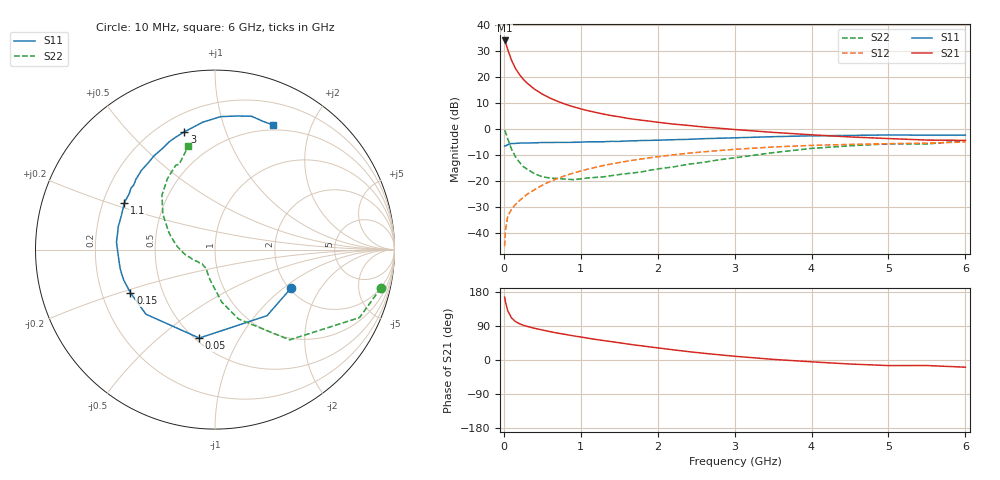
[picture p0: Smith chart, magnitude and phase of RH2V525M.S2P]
! SIEMENS Small Signal Semiconductors
! BFR106
! Si NPN RF Bipolar Junction Transistor in SOT23
! VCE = 2.5 V  IC = 25 mA
! Common Emitter S-Parameters:  August  1996
# GHz  S  MA  R  50
!  f  S11  S21  S12  S22
! GHz  MAG  ANG  MAG  ANG  MAG  ANG  MAG  ANG
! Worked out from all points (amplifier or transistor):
!   36 points, 10 MHz to 6 GHz, reference 50 ohm
!   highest |S21| = 34.2 dB at 10 MHz (marker M1)
!   |S21| within 3 dB of that: start of sweep to 45.07 MHz
!   unconditionally stable (mu >= 1): 324 MHz to 2.431 GHz; 5.267 GHz to end of sweep
!   at 250 MHz: K = 0.94, MSG = 22.9 dB, |S12| = -26.4 dB
!   at 1.4 GHz: K = 1.07, MAG = 7.7 dB, |S12| = -13.5 dB
!   at 6 GHz: K = 1.01, MAG = -0.2 dB, |S12| = -5.0 dB
!   S11 on the Smith chart (normalised r, x): 10 MHz: 2.04, -1.14; 50 MHz: 0.53, -0.69; 150 MHz: 0.32, -0.22; 1.1 GHz: 0.29, +0.22; 3 GHz: 0.30, +0.73; 6 GHz: 0.44, +1.48
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0.01  0.4745 -27.1  51.33 166.2  0.0055 84.5  0.9487 -13.0
0.02  0.4685 -51.8  47.52 154.8  0.0107 71.6  0.8899 -25.2
0.05  0.5006 -100.1  34.47 130.1  0.0206 58.2  0.6524 -50.4
0.1  0.527 -136.9  21.31 111.1  0.0285 53.6  0.4086 -71.2
0.15  0.5292 -152.9  14.9 101.6  0.0349 55.2  0.2949 -82.7
0.2  0.5363 -161.6  11.48 96.1  0.0411 58.2  0.2319 -88.5
0.25  0.5388 -168.0  9.223 91.8  0.0477 60.6  0.1905 -95.0
0.3  0.5384 -172.2  7.746 88.8  0.0548 62.8  0.1692 -99.6
0.4  0.5427 -179.3  5.88 83.6  0.068 65.3  0.1372 -107.6
0.5  0.5505 175.6  4.729 79.2  0.0826 66.3  0.1202 -113.5
0.6  0.5502 170.7  3.967 74.9  0.0972 66.6  0.1136 -118.3
0.7  0.554 166.8  3.427 70.9  0.1115 66.5  0.1113 -123.8
0.9  0.5552 159.9  2.703 63.9  0.1411 65.0  0.1059 -132.5
1.1  0.5688 152.7  2.252 57.3  0.1699 63.1  0.1142 -139.9
1.3  0.5704 146.9  1.941 51.2  0.1987 60.6  0.12 -147.4
1.6  0.5895 138.4  1.621 42.5  0.2396 56.5  0.1384 -157.8
2.2  0.6236 122.9  1.251 26.9  0.3181 47.5  0.1857 -177.4
3  0.678 104.6  0.981 9.9  0.4066 34.9  0.2788 158.5
3.5  0.7134 95.4  0.864 1.7  0.4518 27.2  0.3508 145.9
4.5  0.7542 80.7  0.705 -10.6  0.5059 12.3  0.4756 123.9
5.5  0.7629 69.3  0.614 -14.6  0.5359 2.9  0.5155 112.8
6  0.7659 65.1  0.606 -19.0  0.5645 -4.2  0.5947 104.5
